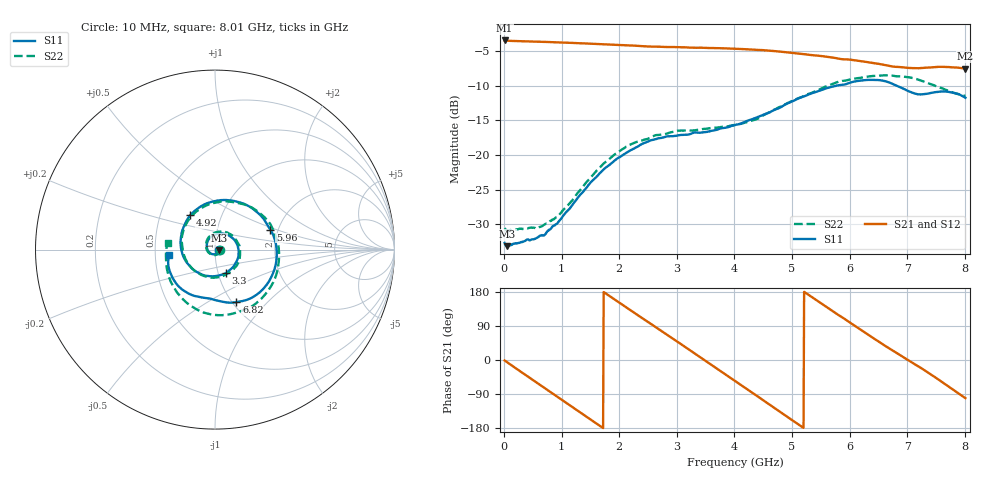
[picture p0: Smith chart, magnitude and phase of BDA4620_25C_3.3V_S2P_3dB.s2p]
!Agilent Technologies,E5071B,MY42404982,A.09.10
!Date: Wed May 06 08:56:36 2026
!Data & Calibration Information:
!Freq	S11:SOLT2(ON)	S21:SOLT2(ON)	S12:SOLT2(ON)	S22:SOLT2(ON)
# Hz S RI R 50
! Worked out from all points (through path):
!   801 points, 10 MHz to 8.01 GHz, reference 50 ohm
!   highest |S21| = -3.44 dB at 10 MHz (marker M1); lowest = -7.5 dB at 8.01 GHz (marker M2)
!   group delay of S21, straight-line fit = 285 ps
!   lowest |S11| = -33.2 dB at 60 MHz (marker M3), VSWR 1.04, Z = 52.2 - j0.313 ohm
!   |S11| at or under -10 dB: start of sweep to 5.761 GHz; 6.821 GHz to end of sweep
!   |S22| runs from -31.0 to -8.5 dB; largest |S21 - S12| = 0.0031
!   S11 on the Smith chart (normalised r, x): 10 MHz: 1.05, -0.00; 3.3 GHz: 1.09, -0.29; 4.92 GHz: 0.71, +0.29; 5.96 GHz: 1.82, +0.46; 6.82 GHz: 1.05, -0.68; 8.01 GHz: 0.59, -0.04
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1e7  0.023 -0.00164  0.6726 -0.0146  0.6732 -0.0147  0.0295 -0.00201
6e7  0.0217 -0.00299  0.6654 -0.0769  0.6669 -0.0779  0.0281 -0.00376
3.7e8  0.0168 -0.0171  0.5142 -0.4191  0.5144 -0.4201  0.0207 -0.0207
7.3e8  -0.0067 -0.0264  0.1491 -0.6389  0.1487 -0.6401  -0.00677 -0.0312
1.03e9  -0.0342 -0.0129  -0.2021 -0.617  -0.203 -0.6177  -0.0371 -0.0153
1.35e9  -0.0462 0.026  -0.502 -0.3999  -0.5023 -0.4003  -0.0506 0.0275
1.64e9  -0.0267 0.067  -0.6265 -0.0942  -0.6274 -0.0945  -0.0312 0.0729
1.93e9  0.0199 0.0897  -0.5828 0.2276  -0.5833 0.228  0.0193 0.0996
2.32e9  0.0934 0.0671  -0.2932 0.5405  -0.2943 0.5413  0.0999 0.0752
2.68e9  0.132 -0.00481  0.0851 0.6  0.0856 0.6005  0.1394 0.00361
3.3e9  0.0608 -0.1319  0.5644 0.1893  0.5656 0.1887  0.0741 -0.1315
3.64e9  -0.0245 -0.1486  0.5683 -0.1688  0.5687 -0.17  -0.0198 -0.1562
4.01e9  -0.1224 -0.11  0.3355 -0.4806  0.3356 -0.4813  -0.1257 -0.107
4.46e9  -0.1909 0.0206  -0.1197 -0.5615  -0.1199 -0.5615  -0.1844 0.0373
4.92e9  -0.1378 0.1913  -0.4794 -0.2741  -0.4799 -0.2743  -0.1013 0.2141
5.35e9  0.0457 0.2763  -0.51 0.1318  -0.5103 0.1324  0.0959 0.2653
5.96e9  0.3081 0.1119  -0.1161 0.4768  -0.1157 0.4781  0.3412 0.0643
6.31e9  0.3357 -0.0949  0.1759 0.4348  0.1771 0.4353  0.3426 -0.1352
6.68e9  0.1945 -0.2735  0.3764 0.2283  0.3779 0.2284  0.2086 -0.3141
6.82e9  0.1198 -0.2928  0.4112 0.1364  0.4124 0.136  0.1296 -0.3471
7.38e9  -0.0915 -0.2635  0.3515 -0.2458  0.3519 -0.2472  -0.1804 -0.2747
8.01e9  -0.2575 -0.0312  -0.0783 -0.4142  -0.0788 -0.4155  -0.2643 0.0368
